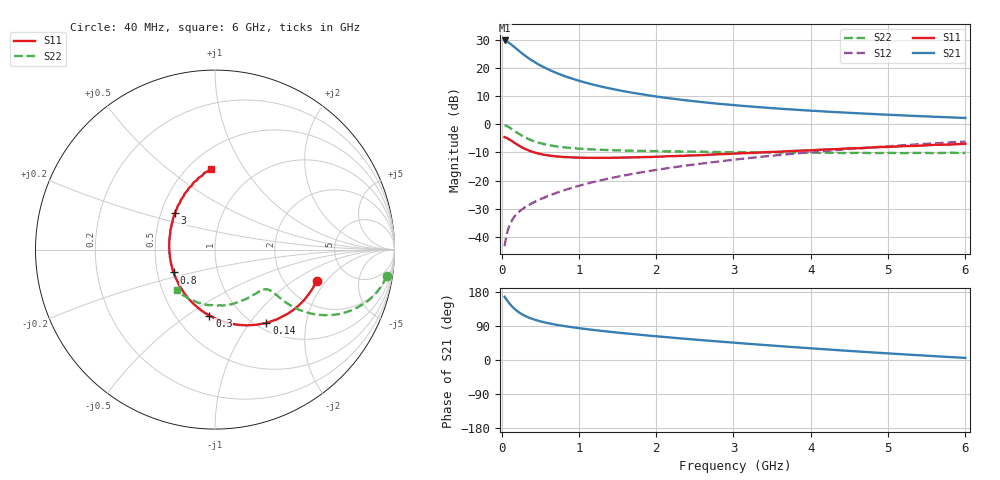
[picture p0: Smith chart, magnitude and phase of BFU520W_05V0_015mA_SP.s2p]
! Filename:  P:\Prog\Test\Noise\ATS_data\Testdata_Net\Run2\BFU520W_APM2013_06_A05_05p0V_015mA_SP_CM01_D.s2p
! Date/Time: Tue 26/Mar/2013 18:01:41
! BFU520W_APM2013_06_A05_05p0V_1to20mA_SP_CM01_Bias7_R.s2p
! MDIF S-parameter v. bias file
! BFU520W_APM2013_06_A05_05p0V_1to20mA_SP_CM01
! Date/time Thu Mar 21 14:22:37 2013
! VAR V_out= 5.0010
! VAR I_out= 14.9950
! VAR V_in= 0.8440
! VAR I_in= 0.1723
! Device data file deembeded for feedlines and parallel
! Original file: \Run2\BFU520W_APM2013_06_A05_05p0V_015mA_SP_CM01_R.s2p
! Feed-files: PR019V01_070313_Feed1.s2p, PR019V01_070313_Feed2.s2p
! Parallel-file: PR019V01_070313_Par.s2p
# MHz S MA R 50
!  Freq-MHz  S11-mag  S11-arg  S21-mag  S21-arg  S12-mag  S12-arg  S22-mag  S22-arg
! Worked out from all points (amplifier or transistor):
!   98 points, 40 MHz to 6 GHz, reference 50 ohm
!   highest |S21| = 29.8 dB at 40 MHz (marker M1)
!   |S21| within 3 dB of that: start of sweep to 194.4 MHz
!   unconditionally stable (mu >= 1): 1.181 GHz to 2.275 GHz
!   at 300 MHz: K = 0.64, MSG = 27.0 dB, |S12| = -29.5 dB
!   at 1.6 GHz: K = 1.01, MAG = 14.2 dB, |S12| = -18.1 dB
!   at 6 GHz: K = 0.87, MSG = 4.2 dB, |S12| = -6.1 dB
!   S11 on the Smith chart (normalised r, x): 40 MHz: 2.96, -1.60; 140 MHz: 1.11, -1.21; 300 MHz: 0.72, -0.61; 800 MHz: 0.61, -0.17; 3 GHz: 0.59, +0.26; 6 GHz: 0.64, +0.73
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40  0.5926 -17.3  30.88 166.9  0.006863 82.8  0.9685 -8.7
50  0.5858 -21.5  30.69 163.8  0.008416 81.2  0.9577 -10.8
60  0.5779 -25.6  29.92 160.8  0.00994 79.5  0.9458 -12.9
90  0.5513 -37.5  28.32 152.5  0.01425 75.4  0.9002 -18.4
120  0.5195 -48.4  26.56 145.0  0.01802 72.1  0.8477 -22.9
140  0.4988 -55.0  25.25 140.6  0.02022 70.3  0.8121 -25.4
180  0.4582 -67.1  22.71 133.0  0.0242 67.6  0.7442 -29.3
220  0.4234 -77.6  20.49 126.5  0.02755 66.2  0.6849 -32.1
260  0.3932 -86.6  18.5 121.2  0.03058 65.4  0.634 -34.0
300  0.3689 -94.9  16.78 116.9  0.03342 65.1  0.5916 -35.2
380  0.3317 -108.6  14.04 109.9  0.03875 65.3  0.5266 -36.4
480  0.303 -122.1  11.57 103.3  0.04532 66.2  0.4728 -36.7
600  0.2818 -135.0  9.536 97.3  0.05329 67.6  0.4304 -36.5
800  0.2628 -151.0  7.328 89.9  0.06689 69.2  0.3921 -36.5
1050  0.2556 -165.5  5.689 82.7  0.08448 70.2  0.3666 -37.2
1500  0.2556 175.6  4.073 72.4  0.1173 70.3  0.3456 -41.1
2050  0.2667 159.2  3.055 61.7  0.1589 68.6  0.3337 -48.0
3000  0.3019 137.8  2.199 45.8  0.2351 63.5  0.3205 -64.0
3100  0.3063 135.7  2.139 44.2  0.2433 62.9  0.3207 -65.7
4100  0.3531 118.9  1.719 29.4  0.3291 55.4  0.3117 -86.4
5200  0.4102 102.9  1.44 15.0  0.4259 45.6  0.308 -112.0
6000  0.4521 92.6  1.297 5.6  0.4935 37.7  0.3104 -132.8
